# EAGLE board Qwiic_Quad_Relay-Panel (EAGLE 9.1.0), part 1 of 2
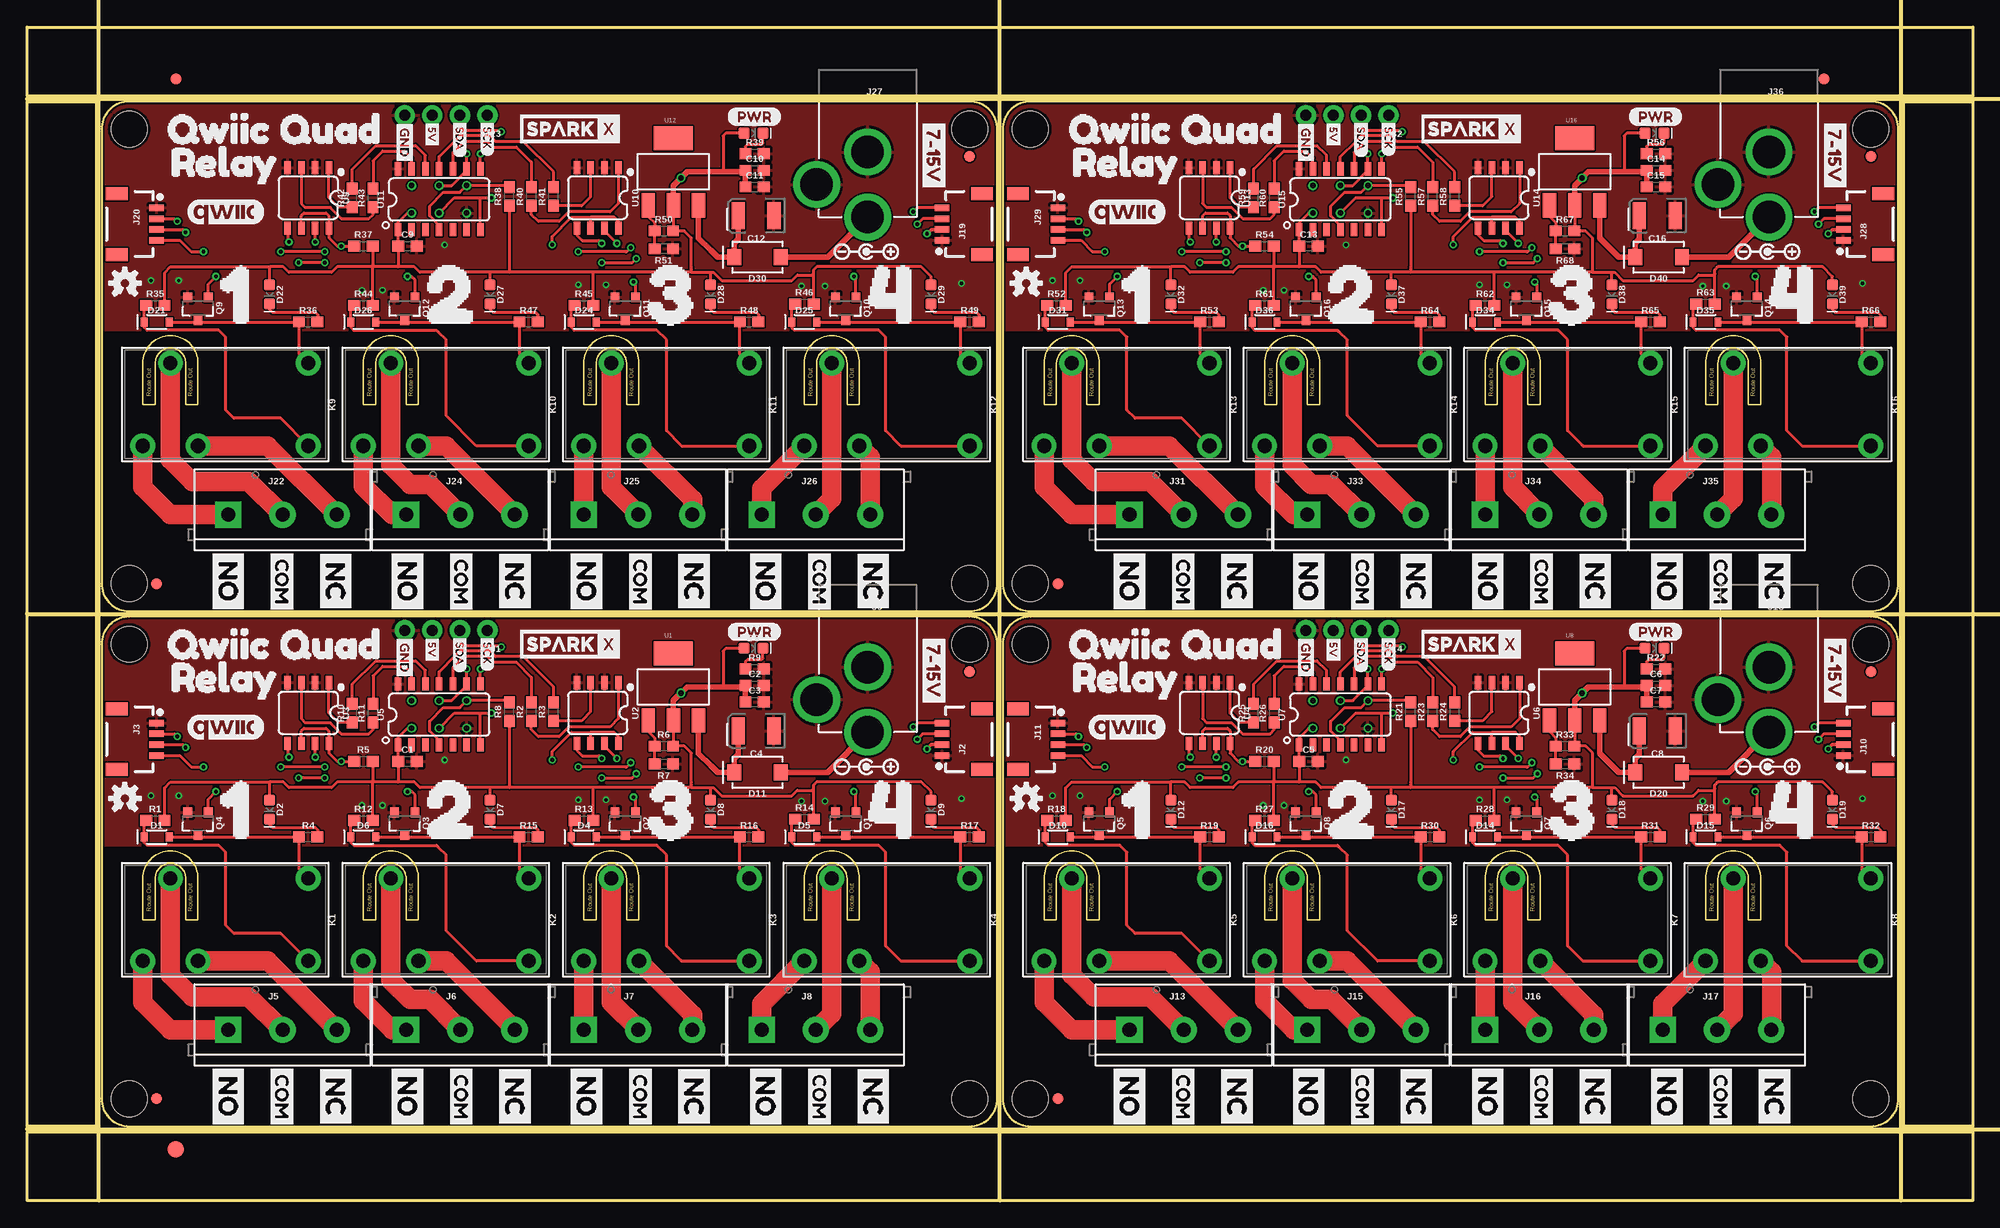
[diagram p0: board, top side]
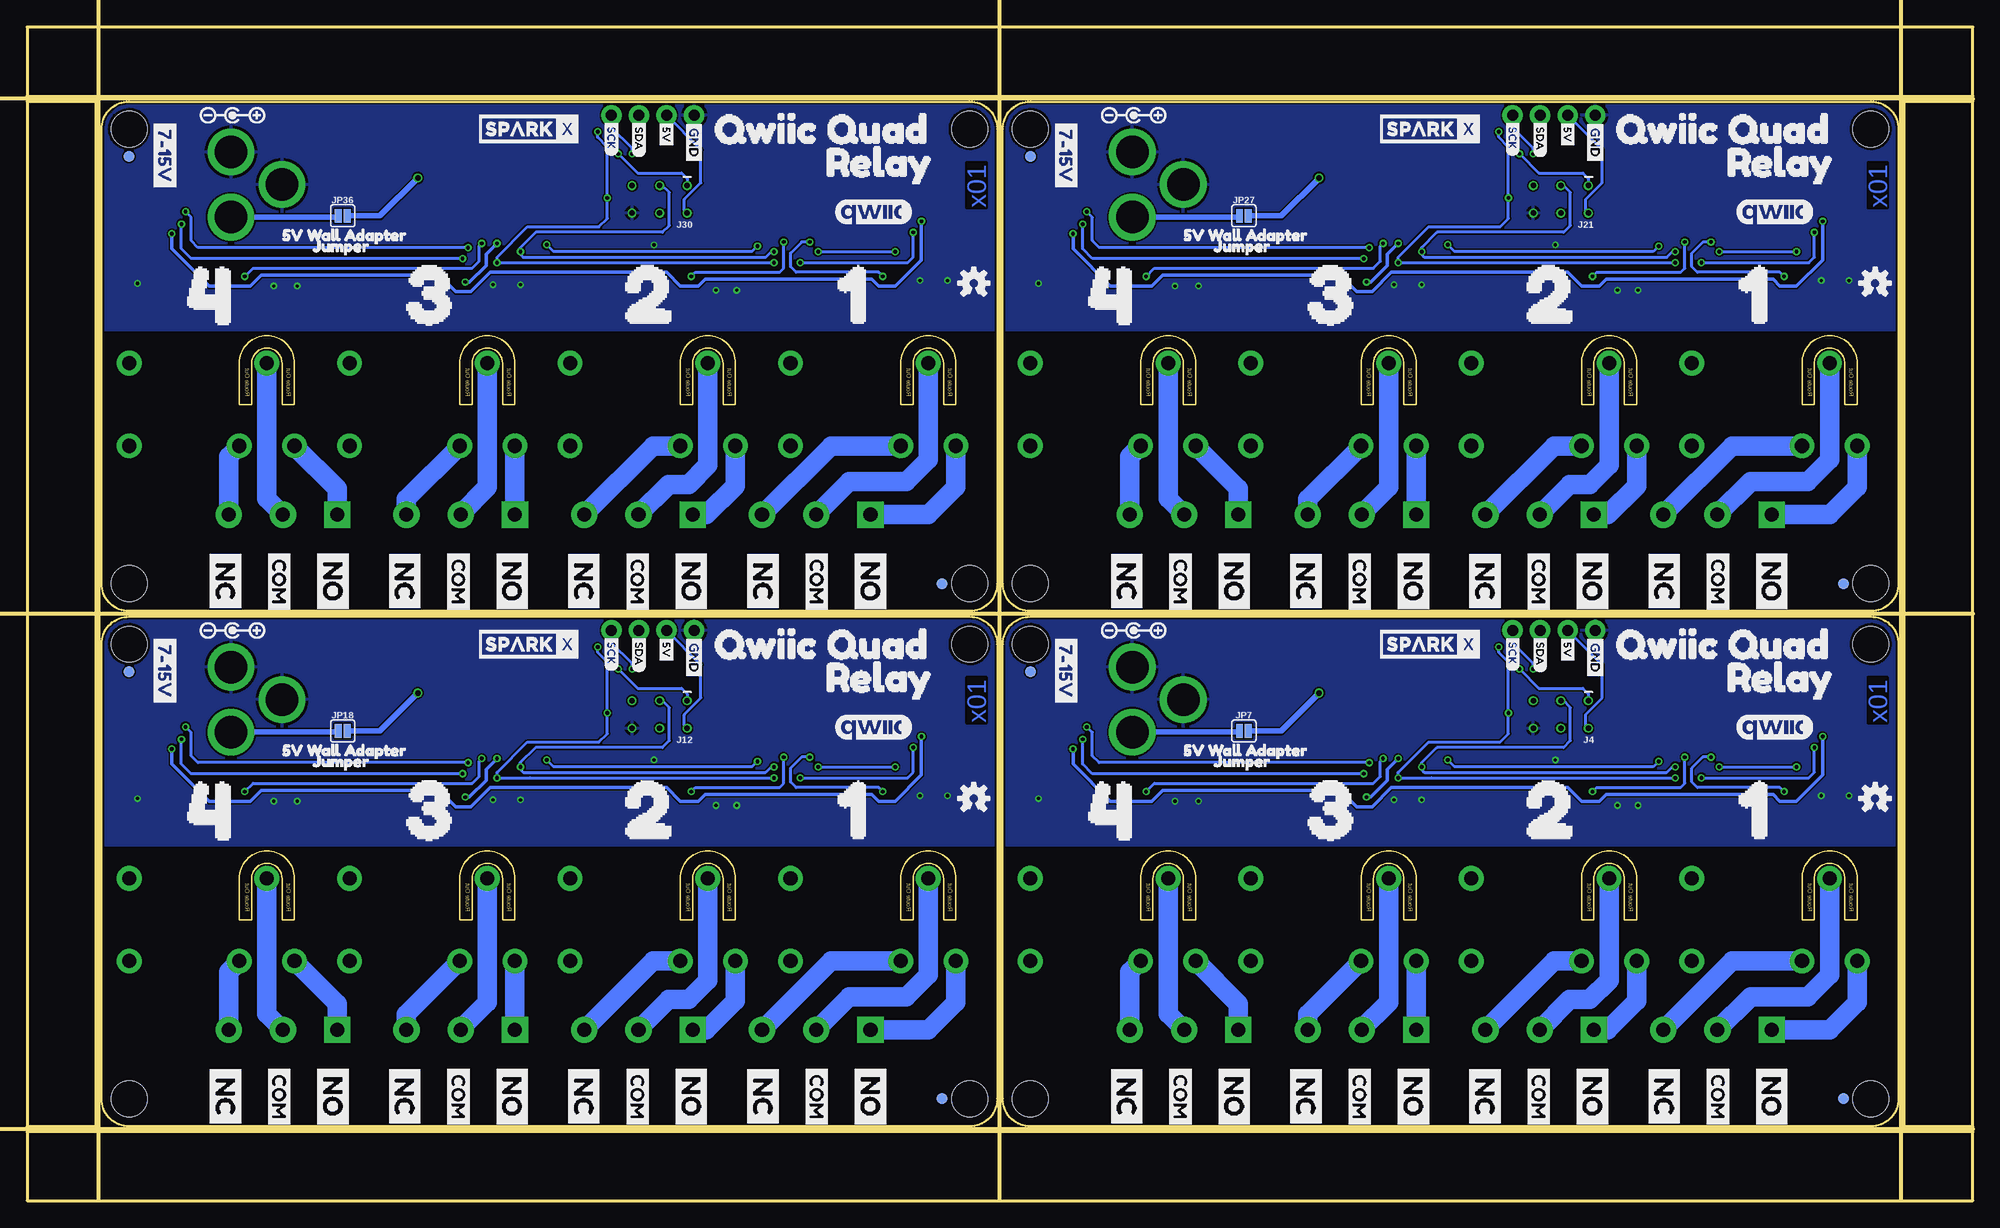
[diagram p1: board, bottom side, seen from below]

Size 179.32 x 108.2 mm. Coordinates in mm from the lower left corner, seen from the top.
Outline: 86.87,53.85 9.4,53.85 arc90 6.86,51.31 6.86,9.4 arc90 9.4,6.86 86.87,6.86 arc90 89.41,9.4 89.41,51.31 arc90 86.87,53.85
Outline: 169.93,53.85 92.46,53.85 arc90 89.92,51.31 89.92,9.4 arc90 92.46,6.86 169.93,6.86 arc90 172.47,9.4 172.47,51.31 arc90 169.93,53.85
Outline: 86.87,101.35 9.4,101.35 arc90 6.86,98.81 6.86,56.9 arc90 9.4,54.36 86.87,54.36 arc90 89.41,56.9 89.41,98.81 arc90 86.87,101.35
Outline: 169.93,101.35 92.46,101.35 arc90 89.92,98.81 89.92,56.9 arc90 92.46,54.36 169.93,54.36 arc90 172.47,56.9 172.47,98.81 arc90 169.93,101.35
Outline: 0,6.35 179.32,6.35 179.32,0 0,0 0,6.35
Outline: 172.97,101.35 179.32,101.35 179.32,6.86 172.97,6.86 172.97,101.35
Outline: 0,108.2 179.32,108.2 179.32,101.85 0,101.85 0,108.2
Outline: 0,101.35 6.35,101.35 6.35,6.86 0,6.86 0,101.35
Copper layers (1*16): Top 0.035mm / dielectric 1.5mm / Bottom 0.035mm
Design rules "SparkFun-2-layer-PCBWay-LIMIT": minimum track width 6mil, minimum drill 0.3mm, track to track 6mil, track to pad 6mil, pad to pad 6mil, via to via 6mil, smd to smd 6mil, copper to edge 6mil, drill to drill 6mil, minimum pad ring 6mil, minimum via ring 6mil, stop-mask expansion 4mil, vias tented up to drill 25mil, thermal gap 10mil
Milling: 166 lines

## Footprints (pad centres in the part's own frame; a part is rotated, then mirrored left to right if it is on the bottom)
0603 = smd 1.1 x 1: 1 -0.85,0; 2 0.85,0
EIA3528 = smd 1.2 x 2.5: A 1.65,0; C -1.65,0
SOD-323 = smd 0.63 x 0.83: A 1.15,0; C -1.15,0
LED-0603 = smd 1 x 1: A -0.877,0; C 0.877,0
SMA-DIODE = smd 1.27 x 1.47: A -2.15,0; C 2.15,0
FIDUCIAL-1X2 = smd 1 x 1: 1 0,0
FIDUCIAL-1.5X3 = smd 1.5 x 1.5: 1 0,0
1X04_NO_SILK = drill 1.016 pad 1.88: 1 0,0; 2 2.54,0; 3 5.08,0; 4 7.62,0
1X04_1MM_RA = smd 0.6 x 1.35: 1 -1.5,0; 2 -0.5,0; 3 0.5,0; 4 1.5,0 | smd 1.2 x 2: NC1 2.8,-3.675; NC2 -2.8,-3.675
2X3_TEST_POINTS = drill 0.508: 1 -2.54,-1.27; 2 -2.54,1.27; 3 0,-1.27; 4 0,1.27; 5 2.54,-1.27; 6 2.54,1.27
SCREWTERMINAL-5MM-3 = drill 1.3 pad 2.413 square: 1 0,0 | drill 1.3 pad 2.413: 2 5,0; 3 10,0
POWER_JACK_PTH = drill 2.997 pad 4.318: GND 0,7.7; GNDBREAK 4.7,10.7; PWR 0,13.7
STAND-OFF = hole 3.302: 0,0
SMT-JUMPER_2_NO_SILK = smd 0.635 x 1.27: 1 -0.406,0; 2 0.406,0
RELAY-JZC = drill 1.3 pad 2.286: 1 3.81,-8.89; 2 -3.81,1.27; 3 -3.81,6.35; 4 3.81,3.81; 5 -3.81,-8.89
SOT23-3 = smd 0.8 x 0.9: 1 -0.95,-1; 2 0.95,-1; 3 0,1.1
SOT223 = smd 1.219 x 2.235: 1 -2.311,-3.099; 2 0,-3.099; 3 2.311,-3.099 | smd 3.6 x 2.2: 4 0,3.099
SO08 = smd 0.6 x 1.2: 1 -1.905,-2.8; 2 -0.635,-2.8; 3 0.635,-2.8; 4 1.905,-2.8; 5 1.905,2.8; 6 0.635,2.8; 7 -0.635,2.8; 8 -1.905,2.8
SO14 = smd 0.6 x 1.2: 1 -3.175,-2.8; 2 -1.905,-2.8; 3 -0.635,-2.8; 4 0.635,-2.8; 5 1.905,-2.8; 6 3.175,-2.8; 7 4.445,-2.8; 8 4.445,2.8; 9 3.175,2.8; 10 1.905,2.8; 11 0.635,2.8; 12 -0.635,2.8; 13 -1.905,2.8; 14 -3.175,2.8

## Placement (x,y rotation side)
C1  0.1uF  [0603]  35.05,40.51 0 top
C2  10uF  [0603]  67.06,47.5 0 top
C3  0.1uF  [0603]  67.06,45.97 0 top
C4  10uF  [EIA3528]  67.18,43.31 180 top
C5  0.1uF  [0603]  118.11,40.51 0 top
C6  10uF  [0603]  150.11,47.5 0 top
C7  0.1uF  [0603]  150.11,45.97 0 top
C8  10uF  [EIA3528]  150.24,43.31 180 top
C9  0.1uF  [0603]  35.05,88.01 0 top
C10  10uF  [0603]  67.06,95 0 top
C11  0.1uF  [0603]  67.06,93.47 0 top
C12  10uF  [EIA3528]  67.18,90.81 180 top
C13  0.1uF  [0603]  118.11,88.01 0 top
C14  10uF  [0603]  150.11,95 0 top
C15  0.1uF  [0603]  150.11,93.47 0 top
C16  10uF  [EIA3528]  150.24,90.81 180 top
D1  1A/23V/620mV  [SOD-323]  11.94,33.53 0 top
D2  WHITE  [LED-0603]  22.35,36.07 270 top
D3  RED  [LED-0603]  66.93,50.93 0 top
D4  1A/23V/620mV  [SOD-323]  51.31,33.53 0 top
D5  1A/23V/620mV  [SOD-323]  71.63,33.53 0 top
D6  1A/23V/620mV  [SOD-323]  30.99,33.53 0 top
D7  BLUE  [LED-0603]  42.67,36.07 270 top
D8  Yellow  [LED-0603]  62.99,36.07 270 top
D9  GREEN  [LED-0603]  83.31,36.07 270 top
D10  1A/23V/620mV  [SOD-323]  95,33.53 0 top
D11  1A/40V/500mV  [SMA-DIODE]  67.31,39.5 180 top
D12  WHITE  [LED-0603]  105.41,36.07 270 top
D13  RED  [LED-0603]  149.99,50.93 0 top
D14  1A/23V/620mV  [SOD-323]  134.37,33.53 0 top
D15  1A/23V/620mV  [SOD-323]  154.69,33.53 0 top
D16  1A/23V/620mV  [SOD-323]  114.05,33.53 0 top
D17  BLUE  [LED-0603]  125.73,36.07 270 top
D18  Yellow  [LED-0603]  146.05,36.07 270 top
D19  GREEN  [LED-0603]  166.37,36.07 270 top
D20  1A/40V/500mV  [SMA-DIODE]  150.37,39.5 180 top
D21  1A/23V/620mV  [SOD-323]  11.94,81.03 0 top
D22  WHITE  [LED-0603]  22.35,83.57 270 top
D23  RED  [LED-0603]  66.93,98.42 0 top
D24  1A/23V/620mV  [SOD-323]  51.31,81.03 0 top
D25  1A/23V/620mV  [SOD-323]  71.63,81.03 0 top
D26  1A/23V/620mV  [SOD-323]  30.99,81.03 0 top
D27  BLUE  [LED-0603]  42.67,83.57 270 top
D28  Yellow  [LED-0603]  62.99,83.57 270 top
D29  GREEN  [LED-0603]  83.31,83.57 270 top
D30  1A/40V/500mV  [SMA-DIODE]  67.31,87 180 top
D31  1A/23V/620mV  [SOD-323]  95,81.03 0 top
D32  WHITE  [LED-0603]  105.41,83.57 270 top
D33  RED  [LED-0603]  149.99,98.42 0 top
D34  1A/23V/620mV  [SOD-323]  134.37,81.03 0 top
D35  1A/23V/620mV  [SOD-323]  154.69,81.03 0 top
D36  1A/23V/620mV  [SOD-323]  114.05,81.03 0 top
D37  BLUE  [LED-0603]  125.73,83.57 270 top
D38  Yellow  [LED-0603]  146.05,83.57 270 top
D39  GREEN  [LED-0603]  166.37,83.57 270 top
D40  1A/40V/500mV  [SMA-DIODE]  150.37,87 180 top
E$1  [FIDUCIAL-1X2]  13.72,103.44 0 top
E$2  [FIDUCIAL-1X2]  165.61,103.44 0 top
E$3  [FIDUCIAL-1.5X3]  13.72,4.76 0 top
J1  [1X04_NO_SILK]  42.42,52.58 180 top
J2  Qwiic Right Angle  [1X04_1MM_RA]  84.33,42.54 90 top
J3  Qwiic Right Angle  [1X04_1MM_RA]  11.94,42.54 270 top
J4  AVR_SPI_PROG_3X2TESTPOINTS  [2X3_TEST_POINTS]  37.97,44.83 180 bottom
J5  [SCREWTERMINAL-5MM-3]  18.54,15.75 0 top
J6  [SCREWTERMINAL-5MM-3]  34.92,15.75 0 top
J7  [SCREWTERMINAL-5MM-3]  51.31,15.75 0 top
J8  [SCREWTERMINAL-5MM-3]  67.69,15.75 0 top
J9  POWER_JACK  [POWER_JACK_PTH]  77.47,56.9 180 top
J10  Qwiic Right Angle  [1X04_1MM_RA]  167.39,42.54 90 top
J11  Qwiic Right Angle  [1X04_1MM_RA]  95,42.54 270 top
J12  AVR_SPI_PROG_3X2TESTPOINTS  [2X3_TEST_POINTS]  121.03,44.83 180 bottom
J13  [SCREWTERMINAL-5MM-3]  101.6,15.75 0 top
J14  [1X04_NO_SILK]  125.48,52.58 180 top
J15  [SCREWTERMINAL-5MM-3]  117.98,15.75 0 top
J16  [SCREWTERMINAL-5MM-3]  134.37,15.75 0 top
J17  [SCREWTERMINAL-5MM-3]  150.75,15.75 0 top
J18  POWER_JACK  [POWER_JACK_PTH]  160.53,56.9 180 top
J19  Qwiic Right Angle  [1X04_1MM_RA]  84.33,90.04 90 top
J20  Qwiic Right Angle  [1X04_1MM_RA]  11.94,90.04 270 top
J21  AVR_SPI_PROG_3X2TESTPOINTS  [2X3_TEST_POINTS]  37.97,92.33 180 bottom
J22  [SCREWTERMINAL-5MM-3]  18.54,63.25 0 top
J23  [1X04_NO_SILK]  42.42,100.08 180 top
J24  [SCREWTERMINAL-5MM-3]  34.92,63.25 0 top
J25  [SCREWTERMINAL-5MM-3]  51.31,63.25 0 top
J26  [SCREWTERMINAL-5MM-3]  67.69,63.25 0 top
J27  POWER_JACK  [POWER_JACK_PTH]  77.47,104.39 180 top
J28  Qwiic Right Angle  [1X04_1MM_RA]  167.39,90.04 90 top
J29  Qwiic Right Angle  [1X04_1MM_RA]  95,90.04 270 top
J30  AVR_SPI_PROG_3X2TESTPOINTS  [2X3_TEST_POINTS]  121.03,92.33 180 bottom
J31  [SCREWTERMINAL-5MM-3]  101.6,63.25 0 top
J32  [1X04_NO_SILK]  125.48,100.08 180 top
J33  [SCREWTERMINAL-5MM-3]  117.98,63.25 0 top
J34  [SCREWTERMINAL-5MM-3]  134.37,63.25 0 top
J35  [SCREWTERMINAL-5MM-3]  150.75,63.25 0 top
J36  POWER_JACK  [POWER_JACK_PTH]  160.53,104.39 180 top
JP1  STAND-OFF  [STAND-OFF]  9.4,9.4 0 top
JP2  FIDUCIAL1X2  [FIDUCIAL-1X2]  86.87,48.77 0 bottom
JP3  STAND-OFF  [STAND-OFF]  9.4,51.31 0 top
JP4  STAND-OFF  [STAND-OFF]  86.87,51.31 0 top
JP5  STAND-OFF  [STAND-OFF]  86.87,9.4 0 top
JP6  FIDUCIAL1X2  [FIDUCIAL-1X2]  11.94,9.4 0 bottom
JP7  JUMPER-SMT_2_NO_SILK  [SMT-JUMPER_2_NO_SILK]  67.18,43.31 0 bottom
JP8  FIDUCIAL1X2  [FIDUCIAL-1X2]  11.94,9.4 0 top
JP9  FIDUCIAL1X2  [FIDUCIAL-1X2]  86.87,48.77 0 top
JP10  STAND-OFF  [STAND-OFF]  92.46,51.31 0 top
JP11  STAND-OFF  [STAND-OFF]  169.93,51.31 0 top
JP12  FIDUCIAL1X2  [FIDUCIAL-1X2]  169.93,48.77 0 bottom
JP13  FIDUCIAL1X2  [FIDUCIAL-1X2]  95,9.4 0 bottom
JP14  STAND-OFF  [STAND-OFF]  92.46,9.4 0 top
JP15  STAND-OFF  [STAND-OFF]  169.93,9.4 0 top
JP16  FIDUCIAL1X2  [FIDUCIAL-1X2]  95,9.4 0 top
JP17  FIDUCIAL1X2  [FIDUCIAL-1X2]  169.93,48.77 0 top
JP18  JUMPER-SMT_2_NO_SILK  [SMT-JUMPER_2_NO_SILK]  150.24,43.31 0 bottom
JP19  STAND-OFF  [STAND-OFF]  9.4,98.81 0 top
JP20  STAND-OFF  [STAND-OFF]  86.87,98.81 0 top
JP21  FIDUCIAL1X2  [FIDUCIAL-1X2]  86.87,96.27 0 bottom
JP22  FIDUCIAL1X2  [FIDUCIAL-1X2]  11.94,56.9 0 bottom
JP23  STAND-OFF  [STAND-OFF]  9.4,56.9 0 top
JP24  STAND-OFF  [STAND-OFF]  86.87,56.9 0 top
JP25  FIDUCIAL1X2  [FIDUCIAL-1X2]  11.94,56.9 0 top
JP26  FIDUCIAL1X2  [FIDUCIAL-1X2]  86.87,96.27 0 top
JP27  JUMPER-SMT_2_NO_SILK  [SMT-JUMPER_2_NO_SILK]  67.18,90.81 0 bottom
JP28  STAND-OFF  [STAND-OFF]  92.46,98.81 0 top
JP29  STAND-OFF  [STAND-OFF]  169.93,98.81 0 top
JP30  FIDUCIAL1X2  [FIDUCIAL-1X2]  169.93,96.27 0 bottom
JP31  FIDUCIAL1X2  [FIDUCIAL-1X2]  95,56.9 0 bottom
JP32  STAND-OFF  [STAND-OFF]  92.46,56.9 0 top
JP33  STAND-OFF  [STAND-OFF]  169.93,56.9 0 top
JP34  FIDUCIAL1X2  [FIDUCIAL-1X2]  95,56.9 0 top
JP35  FIDUCIAL1X2  [FIDUCIAL-1X2]  169.93,96.27 0 top
JP36  JUMPER-SMT_2_NO_SILK  [SMT-JUMPER_2_NO_SILK]  150.24,90.81 0 bottom
K1  RELAY-SPDT-JZC-11F  [RELAY-JZC]  17.02,25.91 90 top
K2  RELAY-SPDT-JZC-11F  [RELAY-JZC]  37.34,25.91 90 top
K3  RELAY-SPDT-JZC-11F  [RELAY-JZC]  57.66,25.91 90 top
K4  RELAY-SPDT-JZC-11F  [RELAY-JZC]  77.98,25.91 90 top
K5  RELAY-SPDT-JZC-11F  [RELAY-JZC]  100.08,25.91 90 top
K6  RELAY-SPDT-JZC-11F  [RELAY-JZC]  120.4,25.91 90 top
K7  RELAY-SPDT-JZC-11F  [RELAY-JZC]  140.72,25.91 90 top
K8  RELAY-SPDT-JZC-11F  [RELAY-JZC]  161.04,25.91 90 top
K9  RELAY-SPDT-JZC-11F  [RELAY-JZC]  17.02,73.41 90 top
K10  RELAY-SPDT-JZC-11F  [RELAY-JZC]  37.34,73.41 90 top
K11  RELAY-SPDT-JZC-11F  [RELAY-JZC]  57.66,73.41 90 top
K12  RELAY-SPDT-JZC-11F  [RELAY-JZC]  77.98,73.41 90 top
K13  RELAY-SPDT-JZC-11F  [RELAY-JZC]  100.08,73.41 90 top
K14  RELAY-SPDT-JZC-11F  [RELAY-JZC]  120.4,73.41 90 top
K15  RELAY-SPDT-JZC-11F  [RELAY-JZC]  140.72,73.41 90 top
K16  RELAY-SPDT-JZC-11F  [RELAY-JZC]  161.04,73.41 90 top
LOGO1  OSHW-LOGOS  [OSHW-LOGO-S]  9.02,37.08 0 top
LOGO2  OSHW-LOGOS  [OSHW-LOGO-S]  92.08,37.08 0 top
LOGO3  OSHW-LOGOS  [OSHW-LOGO-S]  9.02,84.58 0 top
LOGO4  OSHW-LOGOS  [OSHW-LOGO-S]  92.08,84.58 0 top
Q1  600mA/40V  [SOT23-3]  75.44,34.8 180 top
Q2  600mA/40V  [SOT23-3]  55.12,34.8 180 top
Q3  600mA/40V  [SOT23-3]  34.8,34.8 180 top
Q4  600mA/40V  [SOT23-3]  15.75,34.8 180 top
Q5  600mA/40V  [SOT23-3]  98.81,34.8 180 top
Q6  600mA/40V  [SOT23-3]  158.5,34.8 180 top
Q7  600mA/40V  [SOT23-3]  138.18,34.8 180 top
Q8  600mA/40V  [SOT23-3]  117.86,34.8 180 top
Q9  600mA/40V  [SOT23-3]  15.75,82.3 180 top
Q10  600mA/40V  [SOT23-3]  75.44,82.3 180 top
Q11  600mA/40V  [SOT23-3]  55.12,82.3 180 top
Q12  600mA/40V  [SOT23-3]  34.8,82.3 180 top
Q13  600mA/40V  [SOT23-3]  98.81,82.3 180 top
Q14  600mA/40V  [SOT23-3]  158.5,82.3 180 top
Q15  600mA/40V  [SOT23-3]  138.18,82.3 180 top
Q16  600mA/40V  [SOT23-3]  117.86,82.3 180 top
R1  10  [0603]  11.81,35.05 0 top
R2  220  [0603]  46.48,45.08 90 top
R3  220  [0603]  48.51,45.08 90 top
R4  220  [0603]  25.91,33.53 0 top
R5  220  [0603]  30.99,40.51 0 top
R6  240  [0603]  58.67,41.91 0 top
R7  715  [0603]  58.67,40.26 180 top
R8  10K  [0603]  44.45,45.08 90 top
R9  1k  [0603]  67.06,49.02 0 top
R10  220  [0603]  29.97,44.96 90 top
R11  220  [0603]  31.88,44.96 90 top
R12  10  [0603]  30.99,35.05 0 top
R13  10  [0603]  51.31,35.05 0 top
R14  10  [0603]  71.63,35.18 0 top
R15  220  [0603]  46.23,33.53 0 top
R16  220  [0603]  66.55,33.53 0 top
R17  220  [0603]  86.87,33.53 0 top
R18  10  [0603]  94.87,35.05 0 top
R19  220  [0603]  108.97,33.53 0 top
R20  220  [0603]  114.05,40.51 0 top
R21  10K  [0603]  127.51,45.08 90 top
R22  1k  [0603]  150.11,49.02 0 top
R23  220  [0603]  129.54,45.08 90 top
R24  220  [0603]  131.57,45.08 90 top
R25  220  [0603]  113.03,44.96 90 top
R26  220  [0603]  114.94,44.96 90 top
R27  10  [0603]  114.05,35.05 0 top
R28  10  [0603]  134.37,35.05 0 top
R29  10  [0603]  154.69,35.18 0 top
R30  220  [0603]  129.29,33.53 0 top
R31  220  [0603]  149.61,33.53 0 top
R32  220  [0603]  169.93,33.53 0 top
R33  240  [0603]  141.73,41.91 0 top
R34  715  [0603]  141.73,40.26 180 top
R35  10  [0603]  11.81,82.55 0 top
R36  220  [0603]  25.91,81.03 0 top
R37  220  [0603]  30.99,88.01 0 top
R38  10K  [0603]  44.45,92.58 90 top
R39  1k  [0603]  67.06,96.52 0 top
R40  220  [0603]  46.48,92.58 90 top
R41  220  [0603]  48.51,92.58 90 top
R42  220  [0603]  29.97,92.46 90 top
R43  220  [0603]  31.88,92.46 90 top
R44  10  [0603]  30.99,82.55 0 top
R45  10  [0603]  51.31,82.55 0 top
R46  10  [0603]  71.63,82.68 0 top
R47  220  [0603]  46.23,81.03 0 top
R48  220  [0603]  66.55,81.03 0 top
R49  220  [0603]  86.87,81.03 0 top
R50  240  [0603]  58.67,89.41 0 top
R51  715  [0603]  58.67,87.76 180 top
R52  10  [0603]  94.87,82.55 0 top
R53  220  [0603]  108.97,81.03 0 top
R54  220  [0603]  114.05,88.01 0 top
R55  10K  [0603]  127.51,92.58 90 top
R56  1k  [0603]  150.11,96.52 0 top
R57  220  [0603]  129.54,92.58 90 top
R58  220  [0603]  131.57,92.58 90 top
R59  220  [0603]  113.03,92.46 90 top
R60  220  [0603]  114.94,92.46 90 top
R61  10  [0603]  114.05,82.55 0 top
R62  10  [0603]  134.37,82.55 0 top
R63  10  [0603]  154.69,82.68 0 top
R64  220  [0603]  129.29,81.03 0 top
R65  220  [0603]  149.61,81.03 0 top
R66  220  [0603]  169.93,81.03 0 top
R67  240  [0603]  141.73,89.41 0 top
R68  715  [0603]  141.73,87.76 180 top
U1  V_REG_317SMD  [SOT223]  59.56,47.37 0 top
U2  DUAL-OPTOISOLATOR_SOIC8  [SO08]  52.58,44.96 180 top
U3  DUAL-OPTOISOLATOR_SOIC8  [SO08]  25.91,44.96 180 top
U4  DUAL-OPTOISOLATOR_SOIC8  [SO08]  108.97,44.96 180 top
U5  ATTINY84-ARDUINO  [SO14]  37.34,44.83 0 top
U6  DUAL-OPTOISOLATOR_SOIC8  [SO08]  135.64,44.96 180 top
U7  ATTINY84-ARDUINO  [SO14]  120.4,44.83 0 top
U8  V_REG_317SMD  [SOT223]  142.62,47.37 0 top
U9  DUAL-OPTOISOLATOR_SOIC8  [SO08]  25.91,92.46 180 top
U10  DUAL-OPTOISOLATOR_SOIC8  [SO08]  52.58,92.46 180 top
U11  ATTINY84-ARDUINO  [SO14]  37.34,92.33 0 top
U12  V_REG_317SMD  [SOT223]  59.56,94.87 0 top
U13  DUAL-OPTOISOLATOR_SOIC8  [SO08]  108.97,92.46 180 top
U14  DUAL-OPTOISOLATOR_SOIC8  [SO08]  135.64,92.46 180 top
U15  ATTINY84-ARDUINO  [SO14]  120.4,92.33 0 top
U16  V_REG_317SMD  [SOT223]  142.62,94.87 0 top
U$1  [PWR-()-04]  64.52,52.45 0 top
U$2  [20]  32.26,36.07 0 top
U$3  [10]  13.21,36.07 0 top
U$4  [30]  52.58,36.07 0 top
U$5  [40]  72.9,36.07 0 top
U$6  [QWIIC_QUAD_0]  10.67,51.31 0 top
U$7  [RELAY0]  11.05,48.26 0 top
U$8  [SCK-[)-03]  42.42,52.2 270 top
U$9  [GND-03]  34.8,52.2 270 top
U$10  [5V0]  37.34,52.2 270 top
U$11  [SDA0]  39.88,52.2 270 top
U$12  SPARKX-LOGO4  [SPARKX-MEDIUM]  50.04,51.31 0 top
U$13  [OSHW-LOGO-S]  9.02,37.08 0 bottom
U$14  [SPARKX-MEDIUM]  50.04,51.31 0 bottom
U$15  [NO0]  18.54,13.08 270 top
U$16  [COM0]  23.5,12.83 270 top
U$17  [NC0]  28.45,12.95 270 top
U$18  [NO0]  35.05,13.08 270 top
U$19  [COM0]  40,12.83 270 top
U$20  [NC0]  44.96,12.95 270 top
U$21  [NO0]  51.56,13.08 270 top
U$22  [COM0]  56.51,12.83 270 top
U$23  [NC0]  61.47,12.95 270 top
U$24  [NO0]  68.07,13.08 270 top
U$25  [COM0]  73.03,12.83 270 top
U$26  [NC0]  77.98,12.95 270 top
U$27  [NO0]  51.56,13.08 270 bottom
U$28  [COM0]  73.03,12.83 270 bottom
U$29  [NC0]  77.98,12.95 270 bottom
U$30  [NO0]  68.07,13.08 270 bottom
U$31  [COM0]  56.51,12.83 270 bottom
U$32  [NC0]  61.47,12.95 270 bottom
U$33  [NO0]  35.05,13.08 270 bottom
U$34  [COM0]  40,12.83 270 bottom
U$35  [NC0]  44.96,12.95 270 bottom
U$36  [NO0]  18.54,13.08 270 bottom
U$37  [COM0]  23.5,12.83 270 bottom
U$38  [NC0]  28.45,12.95 270 bottom
U$39  [10]  26.16,36.07 0 bottom
U$40  [20]  45.72,36.07 0 bottom
U$41  [30]  65.91,36.07 0 bottom
U$42  [40]  86.11,35.94 0 bottom
U$43  [QWIIC_QUAD_0]  35.18,51.31 0 bottom
U$44  [RELAY0]  24.89,48.26 0 bottom
U$45  [GND-03]  34.8,52.2 270 bottom
U$46  [5V0]  37.34,52.2 270 bottom
U$47  [SDA0]  39.88,52.2 270 bottom
U$48  [SCK-[)-03]  42.42,52.2 270 bottom
U$49  [7#15V0]  83.57,52.45 270 top
U$50  [5V_WALL_ADAPTER0]  73.66,41.53 0 bottom
U$51  [POLARITY_MARKING_CENTER_POSITIVE#JPG]  77.34,40 0 top
U$52  [JUMPER0]  70.87,40.51 0 bottom
U$53  [7#15V0]  83.57,52.45 270 bottom
U$54  [POLARITY_MARKING_CENTER_POSITIVE#JPG]  77.34,52.58 0 bottom
U$55  [QWIIC#JPG]  18.29,43.69 0 top
U$56  [PWR-()-04]  147.57,52.45 0 top
U$57  [QWIIC#JPG]  18.29,43.69 0 bottom
U$58  [20]  115.32,36.07 0 top
U$59  [10]  96.27,36.07 0 top
U$60  [30]  135.64,36.07 0 top
U$61  [40]  155.96,36.07 0 top
U$62  [QWIIC_QUAD_0]  93.73,51.31 0 top
U$63  [RELAY0]  94.11,48.26 0 top
U$64  SPARKX-LOGO4  [SPARKX-MEDIUM]  133.1,51.31 0 top
U$65  [SPARKX-MEDIUM]  133.1,51.31 0 bottom
U$66  [NO0]  101.6,13.08 270 top
U$67  [COM0]  106.55,12.83 270 top
U$68  [NC0]  111.51,12.95 270 top
U$69  [NO0]  118.11,13.08 270 top
U$70  [COM0]  123.06,12.83 270 top
U$71  [NC0]  128.02,12.95 270 top
U$72  [NO0]  134.62,13.08 270 top
U$73  [COM0]  139.57,12.83 270 top
U$74  [NC0]  144.53,12.95 270 top
U$75  [NO0]  151.13,13.08 270 top
U$76  [COM0]  156.08,12.83 270 top
U$77  [NC0]  161.04,12.95 270 top
U$78  [NO0]  134.62,13.08 270 bottom
U$79  [COM0]  156.08,12.83 270 bottom
U$80  [NC0]  161.04,12.95 270 bottom
U$81  [NO0]  151.13,13.08 270 bottom
U$82  [COM0]  139.57,12.83 270 bottom
U$83  [NC0]  144.53,12.95 270 bottom
U$84  [NO0]  118.11,13.08 270 bottom
U$85  [COM0]  123.06,12.83 270 bottom
U$86  [NC0]  128.02,12.95 270 bottom
U$87  [NO0]  101.6,13.08 270 bottom
U$88  [COM0]  106.55,12.83 270 bottom
U$89  [NC0]  111.51,12.95 270 bottom
U$90  [10]  109.22,36.07 0 bottom
U$91  [20]  128.78,36.07 0 bottom
U$92  [30]  148.97,36.07 0 bottom
U$93  [40]  169.16,35.94 0 bottom
U$94  [QWIIC_QUAD_0]  118.24,51.31 0 bottom
U$95  [RELAY0]  107.95,48.26 0 bottom
U$96  [OSHW-LOGO-S]  92.08,37.08 0 bottom
U$97  [7#15V0]  166.62,52.45 270 top
U$98  [SCK-[)-03]  125.48,52.2 270 top
U$99  [GND-03]  117.86,52.2 270 top
U$100  [5V0]  120.4,52.2 270 top
U$101  [SDA0]  122.94,52.2 270 top
U$102  [GND-03]  117.86,52.2 270 bottom
U$103  [5V0]  120.4,52.2 270 bottom
U$104  [SDA0]  122.94,52.2 270 bottom
U$105  [SCK-[)-03]  125.48,52.2 270 bottom
U$106  [POLARITY_MARKING_CENTER_POSITIVE#JPG]  160.4,40 0 top
U$107  [7#15V0]  166.62,52.45 270 bottom
U$108  [POLARITY_MARKING_CENTER_POSITIVE#JPG]  160.4,52.58 0 bottom
U$109  [QWIIC#JPG]  101.35,43.69 0 top
U$110  [QWIIC#JPG]  101.35,43.69 0 bottom
U$111  [5V_WALL_ADAPTER0]  156.72,41.53 0 bottom
U$112  [JUMPER0]  153.92,40.51 0 bottom
U$113  [PWR-()-04]  64.52,99.95 0 top
U$114  [20]  32.26,83.57 0 top
U$115  [10]  13.21,83.57 0 top
U$116  [30]  52.58,83.57 0 top
U$117  [40]  72.9,83.57 0 top
U$118  [QWIIC_QUAD_0]  10.67,98.81 0 top
U$119  [RELAY0]  11.05,95.76 0 top
U$120  SPARKX-LOGO4  [SPARKX-MEDIUM]  50.04,98.81 0 top
U$121  [SPARKX-MEDIUM]  50.04,98.81 0 bottom
U$122  [NO0]  18.54,60.58 270 top
U$123  [COM0]  23.5,60.32 270 top
U$124  [NC0]  28.45,60.45 270 top
U$125  [NO0]  35.05,60.58 270 top
U$126  [COM0]  40,60.32 270 top
U$127  [NC0]  44.96,60.45 270 top
U$128  [NO0]  51.56,60.58 270 top
U$129  [COM0]  56.51,60.32 270 top
U$130  [NC0]  61.47,60.45 270 top
U$131  [NO0]  68.07,60.58 270 top
U$132  [COM0]  73.03,60.32 270 top
U$133  [NC0]  77.98,60.45 270 top
U$134  [NO0]  51.56,60.58 270 bottom
U$135  [COM0]  73.03,60.32 270 bottom
U$136  [NC0]  77.98,60.45 270 bottom
U$137  [NO0]  68.07,60.58 270 bottom
U$138  [COM0]  56.51,60.32 270 bottom
U$139  [NC0]  61.47,60.45 270 bottom
U$140  [NO0]  35.05,60.58 270 bottom
U$141  [COM0]  40,60.32 270 bottom
U$142  [NC0]  44.96,60.45 270 bottom
U$143  [NO0]  18.54,60.58 270 bottom
U$144  [COM0]  23.5,60.32 270 bottom
U$145  [NC0]  28.45,60.45 270 bottom
U$146  [10]  26.16,83.57 0 bottom
U$147  [20]  45.72,83.57 0 bottom
U$148  [30]  65.91,83.57 0 bottom
U$149  [40]  86.11,83.44 0 bottom
U$150  [QWIIC_QUAD_0]  35.18,98.81 0 bottom
U$151  [RELAY0]  24.89,95.76 0 bottom
U$152  [OSHW-LOGO-S]  9.02,84.58 0 bottom
U$153  [7#15V0]  83.57,99.95 270 top
U$154  [SCK-[)-03]  42.42,99.7 270 top
U$155  [GND-03]  34.8,99.7 270 top
U$156  [5V0]  37.34,99.7 270 top
U$157  [SDA0]  39.88,99.7 270 top
U$158  [GND-03]  34.8,99.7 270 bottom
U$159  [5V0]  37.34,99.7 270 bottom
U$160  [SDA0]  39.88,99.7 270 bottom
U$161  [SCK-[)-03]  42.42,99.7 270 bottom
U$162  [POLARITY_MARKING_CENTER_POSITIVE#JPG]  77.34,87.5 0 top
U$163  [7#15V0]  83.57,99.95 270 bottom
U$164  [POLARITY_MARKING_CENTER_POSITIVE#JPG]  77.34,100.08 0 bottom
U$165  [QWIIC#JPG]  18.29,91.19 0 top
U$166  [QWIIC#JPG]  18.29,91.19 0 bottom
U$167  [5V_WALL_ADAPTER0]  73.66,89.03 0 bottom
U$168  [JUMPER0]  70.87,88.01 0 bottom
U$169  [PWR-()-04]  147.57,99.95 0 top
U$170  [20]  115.32,83.57 0 top
U$171  [10]  96.27,83.57 0 top
U$172  [30]  135.64,83.57 0 top
U$173  [40]  155.96,83.57 0 top
U$174  [QWIIC_QUAD_0]  93.73,98.81 0 top
U$175  [RELAY0]  94.11,95.76 0 top
U$176  SPARKX-LOGO4  [SPARKX-MEDIUM]  133.1,98.81 0 top
U$177  [SPARKX-MEDIUM]  133.1,98.81 0 bottom
U$178  [NO0]  101.6,60.58 270 top
U$179  [COM0]  106.55,60.32 270 top
U$180  [NC0]  111.51,60.45 270 top
U$181  [NO0]  118.11,60.58 270 top
U$182  [COM0]  123.06,60.32 270 top
U$183  [NC0]  128.02,60.45 270 top
U$184  [NO0]  134.62,60.58 270 top
U$185  [COM0]  139.57,60.32 270 top
U$186  [NC0]  144.53,60.45 270 top
U$187  [NO0]  151.13,60.58 270 top
U$188  [COM0]  156.08,60.32 270 top
U$189  [NC0]  161.04,60.45 270 top
U$190  [NO0]  134.62,60.58 270 bottom
U$191  [COM0]  156.08,60.32 270 bottom
U$192  [NC0]  161.04,60.45 270 bottom
U$193  [NO0]  151.13,60.58 270 bottom
U$194  [COM0]  139.57,60.32 270 bottom
U$195  [NC0]  144.53,60.45 270 bottom
U$196  [NO0]  118.11,60.58 270 bottom
U$197  [COM0]  123.06,60.32 270 bottom
U$198  [NC0]  128.02,60.45 270 bottom
U$199  [NO0]  101.6,60.58 270 bottom
U$200  [COM0]  106.55,60.32 270 bottom
U$201  [NC0]  111.51,60.45 270 bottom
U$202  [10]  109.22,83.57 0 bottom
U$203  [20]  128.78,83.57 0 bottom
U$204  [30]  148.97,83.57 0 bottom
U$205  [40]  169.16,83.44 0 bottom
U$206  [QWIIC_QUAD_0]  118.24,98.81 0 bottom
U$207  [RELAY0]  107.95,95.76 0 bottom
U$208  [OSHW-LOGO-S]  92.08,84.58 0 bottom
U$209  [7#15V0]  166.62,99.95 270 top
U$210  [SCK-[)-03]  125.48,99.7 270 top
U$211  [GND-03]  117.86,99.7 270 top
U$212  [5V0]  120.4,99.7 270 top
U$213  [SDA0]  122.94,99.7 270 top
U$214  [GND-03]  117.86,99.7 270 bottom
U$215  [5V0]  120.4,99.7 270 bottom
U$216  [SDA0]  122.94,99.7 270 bottom
U$217  [SCK-[)-03]  125.48,99.7 270 bottom
U$218  [POLARITY_MARKING_CENTER_POSITIVE#JPG]  160.4,87.5 0 top
U$219  [7#15V0]  166.62,99.95 270 bottom
U$220  [POLARITY_MARKING_CENTER_POSITIVE#JPG]  160.4,100.08 0 bottom
U$221  [QWIIC#JPG]  101.35,91.19 0 top
U$222  [QWIIC#JPG]  101.35,91.19 0 bottom
U$223  [5V_WALL_ADAPTER0]  156.72,89.03 0 bottom
U$224  [JUMPER0]  153.92,88.01 0 bottom

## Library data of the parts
C1 C3 C5 C7 C9 C11 C13 C15 = SparkFun-Capacitors; PROD_ID: CAP-00810
C2 C6 C10 C14 = SparkFun-Capacitors; PROD_ID: CAP-11015
C4 C8 C12 C16 = SparkFun-Capacitors; PROD_ID: CAP-08063
D1 D4-D6 D10 D14-D16 D21 D24-D26 D31 D34-D36 = SparkFun-DiscreteSemi; PROD_ID: DIO-11623
D2 D12 D22 D32 = SparkFun-LED; PROD_ID: DIO-09004
D3 D13 D23 D33 = SparkFun-LED; PROD_ID: DIO-00819
D7 D17 D27 D37 = SparkFun-LED; PROD_ID: DIO-08575
D8 D18 D28 D38 = SparkFun-LED; PROD_ID: DIO-09003
D9 D19 D29 D39 = SparkFun-LED; PROD_ID: DIO-00821
D11 D20 D30 D40 = SparkFun-DiscreteSemi; PROD_ID: DIO-08053
E$1 E$2 JP2 JP6 JP8 JP9 JP12 JP13 JP16 JP17 JP21 JP22 JP25 JP26 JP30 JP31 JP34 JP35 LOGO1-LOGO4 U$13 U$96 U$152 U$208 = SparkFun-Aesthetics
E$3 = SparkFun-Retired
J1 J14 J23 J32 = SparkFun-Connectors; PROD_ID: CONN-09696
J2 J3 J10 J11 J19 J20 J28 J29 = SparkFun-Connectors; PROD_ID: CONN-13694
J4 J12 J21 J30 = SparkFun-Connectors
J5-J8 J13 J15-J17 J22 J24-J26 J31 J33-J35 = SparkFun-Connectors; PROD_ID: CONN-10134; SF_SKU: PRT-08433
J9 J18 J27 J36 = SparkFun-Connectors; PROD_ID: CONN-08197
JP1 JP3-JP5 JP10 JP11 JP14 JP15 JP19 JP20 JP23 JP24 JP28 JP29 JP32 JP33 = SparkFun
JP7 JP18 JP27 JP36 = SparkFun-Jumpers
K1-K16 = SparkFun-Electromechanical; PROD_ID: COMP-09533; SF_SKU: COM-00100
Q1-Q16 = SparkFun-DiscreteSemi; PROD_ID: TRANS-08049
R1 R12-R14 R18 R27-R29 R35 R44-R46 R52 R61-R63 = SparkFun-Resistors; PROD_ID: RES-07871
R2-R5 R10 R11 R15-R17 R19 R20 R23-R26 R30-R32 R36 R37 R40-R43 R47-R49 R53 R54 R57-R60 R64-R66 = SparkFun-Resistors; PROD_ID: RES-07861
R6 R33 R50 R67 = SparkFun-Resistors; PROD_ID: RES-07849
R7 R34 R51 R68 = SparkFun-Resistors; PROD_ID: RES-07850
R8 R9 R21 R22 R38 R39 R55 R56 = SparkFun-Resistors; PROD_ID: RES-00818
U1 U8 U12 U16 = SparkFun-IC-Power
U2-U4 U6 U9 U10 U13 U14 = SparkFun-DiscreteSemi; PROD_ID: IC-09076
U5 U7 U11 U15 = SparkFun-IC-Microcontroller; PROD_ID: IC-11285
U$1 U$8 U$9 U$45 U$48 U$56 U$98 U$99 U$102 U$105 U$113 U$154 U$155 U$158 U$161 U$169 U$210 U$211 U$214 U$217 = Labels
U$2 U$40 U$58 U$91 U$114 U$147 U$170 U$203 = 2
U$3 U$39 U$59 U$90 U$115 U$146 U$171 U$202 = 1
U$4 U$41 U$60 U$92 U$116 U$148 U$172 U$204 = 3
U$5 U$42 U$61 U$93 U$117 U$149 U$173 U$205 = 4
U$6 U$43 U$62 U$94 U$118 U$150 U$174 U$206 = Quad
U$7 U$44 U$63 U$95 U$119 U$151 U$175 U$207 = relay
U$10 U$46 U$100 U$103 U$156 U$159 U$212 U$215 = 5V
U$11 U$47 U$101 U$104 U$157 U$160 U$213 U$216 = SDA
U$12 U$14 U$64 U$65 U$120 U$121 U$176 U$177 = SparkX
U$15 U$18 U$21 U$24 U$27 U$30 U$33 U$36 U$66 U$69 U$72 U$75 U$78 U$81 U$84 U$87 U$122 U$125 U$128 U$131 U$134 U$137 U$140 U$143 U$178 U$181 U$184 U$187 U$190 U$193 U$196 U$199 = NO
U$16 U$19 U$22 U$25 U$28 U$31 U$34 U$37 U$67 U$70 U$73 U$76 U$79 U$82 U$85 U$88 U$123 U$126 U$129 U$132 U$135 U$138 U$141 U$144 U$179 U$182 U$185 U$188 U$191 U$194 U$197 U$200 = COM
U$17 U$20 U$23 U$26 U$29 U$32 U$35 U$38 U$68 U$71 U$74 U$77 U$80 U$83 U$86 U$89 U$124 U$127 U$130 U$133 U$136 U$139 U$142 U$145 U$180 U$183 U$186 U$189 U$192 U$195 U$198 U$201 = NC
U$49 U$53 U$97 U$107 U$153 U$163 U$209 U$219 = 7-15V
U$50 U$111 U$167 U$223 = 5V Wall Adapter
U$51 U$54 U$106 U$108 U$162 U$164 U$218 U$220 = Polarity_marking_center_positive#jpg
U$52 U$112 U$168 U$224 = jumper
U$55 U$57 U$109 U$110 U$165 U$166 U$221 U$222 = qwiic_copyrighted_logo_medium

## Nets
3.3V: J2.2 J3.2
3.3V1: J10.2 J11.2
3.3V2: J19.2 J20.2
3.3V3: J28.2 J29.2
5V: C1.1 C2.1 C3.1 D2.A D3.A D7.A D8.A D9.A J1.3 J4.2 JP7.2 R1.2 R5.2 R6.2 R8.1 R12.2 R13.2 R14.2 U1.2 U5.1
5V1: C5.1 C6.1 C7.1 D12.A D13.A D17.A D18.A D19.A J12.2 J14.3 JP18.2 R18.2 R20.2 R21.1 R27.2 R28.2 R29.2 R33.2 U7.1 U8.2
5V2: C9.1 C10.1 C11.1 D22.A D23.A D27.A D28.A D29.A J21.2 J23.3 JP27.2 R35.2 R37.2 R38.1 R44.2 R45.2 R46.2 R50.2 U11.1 U12.2
5V3: C13.1 C14.1 C15.1 D32.A D33.A D37.A D38.A D39.A J30.2 J32.3 JP36.2 R52.2 R54.2 R55.1 R61.2 R62.2 R63.2 R67.2 U15.1 U16.2
!RESET: J4.5 R8.2 U5.4
!RESET1: J12.5 R21.2 U7.4
!RESET2: J21.5 R38.2 U11.4
!RESET3: J30.5 R55.2 U15.4
COM1: J5.2 K1.4
COM2: J6.2 K2.4
COM3: J7.2 K3.4
COM4: J8.2 K4.4
COM5: J13.2 K5.4
COM6: J15.2 K6.4
COM7: J16.2 K7.4
COM8: J17.2 K8.4
COM9: J22.2 K9.4
COM10: J24.2 K10.4
COM11: J25.2 K11.4
COM12: J26.2 K12.4
COM13: J31.2 K13.4
COM14: J33.2 K14.4
COM15: J34.2 K15.4
COM16: J35.2 K16.4
GND: C1.2 C2.2 C3.2 C4.C J1.4 J2.1 J3.1 J4.6 J9.GND J9.GNDBREAK Q1.2 Q2.2 Q3.2 Q4.2 R7.1 R9.2 U2.2 U2.4 U3.2 U3.4 U5.14
GND1: C5.2 C6.2 C7.2 C8.C J10.1 J11.1 J12.6 J14.4 J18.GND J18.GNDBREAK Q5.2 Q6.2 Q7.2 Q8.2 R22.2 R34.1 U4.2 U4.4 U6.2 U6.4 U7.14
GND2: C9.2 C10.2 C11.2 C12.C J19.1 J20.1 J21.6 J23.4 J27.GND J27.GNDBREAK Q9.2 Q10.2 Q11.2 Q12.2 R39.2 R51.1 U9.2 U9.4 U10.2 U10.4 U11.14
GND3: C13.2 C14.2 C15.2 C16.C J28.1 J29.1 J30.6 J32.4 J36.GND J36.GNDBREAK Q13.2 Q14.2 Q15.2 Q16.2 R56.2 R68.1 U13.2 U13.4 U14.2 U14.4 U15.14
MISO: J4.1 U5.8
MISO1: J12.1 U7.8
MISO2: J21.1 U11.8
MISO3: J30.1 U15.8
N$1: D6.C K2.5 R12.1
N$2: D1.A K1.1 Q4.3 R4.1
N$3: R11.1 U3.3
N$4: C4.A D11.C U1.3
N$5: R10.1 U3.1
N$6: R5.1 U2.6 U2.8 U3.6 U3.8
N$7: D1.C K1.5 R1.1
N$8: D2.C R4.2
N$9: R2.1 U2.1
N$10: D10.A K5.1 Q5.3 R19.1
N$11: R3.1 U2.3
N$12: D6.A K2.1 Q3.3 R15.1
N$13: D3.C R9.1
N$14: D4.C K3.5 R13.1
N$15: D4.A K3.1 Q2.3 R16.1
N$16: D5.C K4.5 R14.1
N$17: D5.A K4.1 Q1.3 R17.1
N$18: D10.C K5.5 R18.1
N$19: R6.1 R7.2 U1.1
N$20: D9.C R17.2
N$21: D8.C R16.2
N$22: D7.C R15.2
N$23: D12.C R19.2
N$24: D13.C R22.1
N$25: R26.1 U4.3
N$26: R25.1 U4.1
N$27: R20.1 U4.6 U4.8 U6.6 U6.8
N$28: R23.1 U6.1
N$29: R24.1 U6.3
N$30: D16.C K6.5 R27.1
N$31: D16.A K6.1 Q8.3 R30.1
N$32: D14.C K7.5 R28.1
N$33: D14.A K7.1 Q7.3 R31.1
N$34: D15.C K8.5 R29.1
N$35: D15.A K8.1 Q6.3 R32.1
N$36: D19.C R32.2
N$37: D18.C R31.2
N$38: D17.C R30.2
N$39: R33.1 R34.2 U8.1
N$40: C8.A D20.C U8.3
N$41: D21.A K9.1 Q9.3 R36.1
N$42: D21.C K9.5 R35.1
N$43: D22.C R36.2
N$44: D23.C R39.1
N$45: R43.1 U9.3
N$46: R42.1 U9.1
N$47: R37.1 U9.6 U9.8 U10.6 U10.8
N$48: R40.1 U10.1
N$49: R41.1 U10.3
N$50: D26.C K10.5 R44.1
N$51: D26.A K10.1 Q12.3 R47.1
N$52: D24.C K11.5 R45.1
N$53: D24.A K11.1 Q11.3 R48.1
N$54: D25.C K12.5 R46.1
N$55: D25.A K12.1 Q10.3 R49.1
N$56: D29.C R49.2
N$57: D28.C R48.2
N$58: D27.C R47.2
N$59: R50.1 R51.2 U12.1
N$60: C12.A D30.C U12.3
N$61: D31.A K13.1 Q13.3 R53.1
N$62: D31.C K13.5 R52.1
N$63: D32.C R53.2
N$64: D33.C R56.1
N$65: R60.1 U13.3
N$66: R59.1 U13.1
N$67: R54.1 U13.6 U13.8 U14.6 U14.8
N$68: R57.1 U14.1
N$69: R58.1 U14.3
N$70: D36.C K14.5 R61.1
N$71: D36.A K14.1 Q16.3 R64.1
N$72: D34.C K15.5 R62.1
N$73: D34.A K15.1 Q15.3 R65.1
N$74: D35.C K16.5 R63.1
N$75: D35.A K16.1 Q14.3 R66.1
N$76: D39.C R66.2
N$77: D38.C R65.2
N$78: D37.C R64.2
N$79: R67.1 R68.2 U16.1
N$80: C16.A D40.C U16.3
NC1: J5.3 K1.2
NC2: J6.3 K2.2
NC3: J7.3 K3.2
NC4: J8.3 K4.2
NC5: J13.3 K5.2
NC6: J15.3 K6.2
NC7: J16.3 K7.2
NC8: J17.3 K8.2
NC9: J22.3 K9.2
NC10: J24.3 K10.2
NC11: J25.3 K11.2
NC12: J26.3 K12.2
NC13: J31.3 K13.2
NC14: J33.3 K14.2
NC15: J34.3 K15.2
NC16: J35.3 K16.2
NO1: J5.1 K1.3
NO2: J6.1 K2.3
NO3: J7.1 K3.3
NO4: J8.1 K4.3
NO5: J13.1 K5.3
NO6: J15.1 K6.3
NO7: J16.1 K7.3
NO8: J17.1 K8.3
NO9: J22.1 K9.3
NO10: J24.1 K10.3
NO11: J25.1 K11.3
NO12: J26.1 K12.3
NO13: J31.1 K13.3
NO14: J33.1 K14.3
NO15: J34.1 K15.3
NO16: J35.1 K16.3
OPTO_1: Q4.1 U3.5
OPTO_2: Q3.1 U3.7
OPTO_3: Q2.1 U2.5
OPTO_4: Q1.1 U2.7
OPTO_5: Q5.1 U4.5
OPTO_6: Q8.1 U4.7
OPTO_7: Q7.1 U6.5
OPTO_8: Q6.1 U6.7
OPTO_9: Q9.1 U9.5
OPTO_10: Q12.1 U9.7
OPTO_11: Q11.1 U10.5
OPTO_12: Q10.1 U10.7
OPTO_13: Q13.1 U13.5
OPTO_14: Q16.1 U13.7
OPTO_15: Q15.1 U14.5
OPTO_16: Q14.1 U14.7
RELAY_CTRL1: R2.2 U5.10
RELAY_CTRL2: R3.2 U5.11
RELAY_CTRL3: R10.2 U5.12
RELAY_CTRL4: R11.2 U5.13
RELAY_CTRL5: R23.2 U7.10
RELAY_CTRL6: R24.2 U7.11
RELAY_CTRL7: R25.2 U7.12
RELAY_CTRL8: R26.2 U7.13
RELAY_CTRL9: R40.2 U11.10
RELAY_CTRL10: R41.2 U11.11
RELAY_CTRL11: R42.2 U11.12
RELAY_CTRL12: R43.2 U11.13
RELAY_CTRL13: R57.2 U15.10
RELAY_CTRL14: R58.2 U15.11
RELAY_CTRL15: R59.2 U15.12
RELAY_CTRL16: R60.2 U15.13
SCL/SCK: J1.1 J2.4 J3.4 J4.3 U5.9
SCL/SCK1: J10.4 J11.4 J12.3 J14.1 U7.9
SCL/SCK2: J19.4 J20.4 J21.3 J23.1 U11.9
SCL/SCK3: J28.4 J29.4 J30.3 J32.1 U15.9
SDA/MOSI: J1.2 J2.3 J3.3 J4.4 U5.7
SDA/MOSI1: J10.3 J11.3 J12.4 J14.2 U7.7
SDA/MOSI2: J19.3 J20.3 J21.4 J23.2 U11.7
SDA/MOSI3: J28.3 J29.3 J30.4 J32.2 U15.7
VIN: D11.A J9.PWR JP7.1
VIN1: D20.A J18.PWR JP18.1
VIN2: D30.A J27.PWR JP27.1
VIN3: D40.A J36.PWR JP36.1

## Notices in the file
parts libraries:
SparkFun-Capacitors: Licensing: Creative Commons ShareAlike 4.0 International - https://creativecommons.org/licenses/by-sa/4.0
